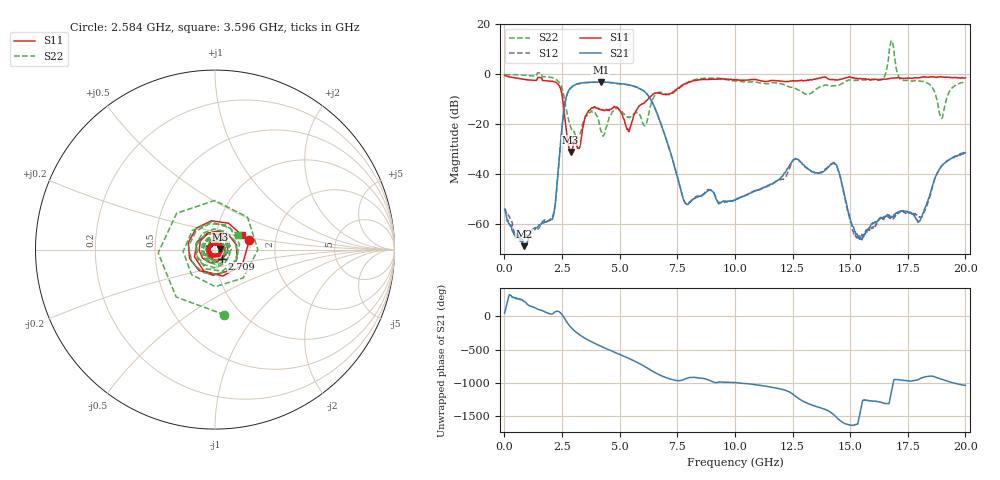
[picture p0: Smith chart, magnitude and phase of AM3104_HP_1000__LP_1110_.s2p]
!Created with skrf (http://scikit-rf.org).
# Hz S RI R 50.0
!freq ReS11 ImS11 ReS21 ImS21 ReS12 ImS12 ReS22 ImS22
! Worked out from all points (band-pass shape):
!   1601 points, 10 MHz to 20 GHz, reference 50 ohm
!   highest |S21| = -2.97 dB at 4.183 GHz (marker M1); lowest = -68.7 dB at 859.6 MHz (marker M2)
!   |S21| within 3 dB of the highest: 2.824 GHz to 5.941 GHz (3.117 GHz wide, 71.1 % of centre)
!   lowest |S11| = -31.0 dB at 2.871 GHz (marker M3), VSWR 1.06, Z = 52.9 + j0.371 ohm
!   |S11| at or under -10 dB: 2.53 GHz to 6.218 GHz (3.688 GHz wide, 84.3 % of centre)
!   |S22| runs from -25.6 to 13.6 dB; largest |S21 - S12| = 0.078
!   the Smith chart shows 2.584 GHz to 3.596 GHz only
!   S11 on the Smith chart (normalised r, x): 2.584 GHz: 1.46, +0.16; 2.709 GHz: 1.08, -0.11; 3.596 GHz: 1.33, +0.22
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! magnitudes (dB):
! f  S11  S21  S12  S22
! 10 MHz  -0.4  -54.0  -53.6  -0.1
! 859.6 MHz  -2.0  -68.7  -65.8  -0.2
! 2.096 GHz  -2.8  -57.6  -56.5  -1.4
! 2.584 GHz  -14.1  -14.3  -14.3  -8.7
! 2.709 GHz  -23.8  -8.3  -8.3  -15.0
! 2.871 GHz  -31.0  -5.4  -5.5  -20.9
! 3.346 GHz  -24.9  -3.4  -3.5  -22.0
! 3.596 GHz  -15.4  -3.2  -3.3  -16.3
! 4.183 GHz  -14.1  -3.0  -3.0  -22.4
! 5.382 GHz  -22.6  -4.1  -4.2  -17.1
! 6.107 GHz  -11.0  -7.1  -7.1  -20.5
! 6.682 GHz  -7.3  -17.0  -17.0  -7.2
! 7.869 GHz  -3.7  -51.6  -51.6  -3.6
! 10.01 GHz  -2.2  -50.4  -50.1  -2.7
! 12.6 GHz  -2.6  -33.8  -33.9  -5.4
! 13.34 GHz  -2.2  -38.9  -38.9  -7.3
! 14.37 GHz  -2.1  -35.9  -36.2  -4.5
! 15.43 GHz  -1.6  -65.9  -64.6  -2.3
! 16.68 GHz  -1.7  -56.4  -57.2  7.3
! 18.03 GHz  -1.4  -58.6  -57.1  -2.7
! 18.95 GHz  -0.9  -36.9  -36.9  -17.3
! 20 GHz  -1.4  -31.4  -30.8  -2.8
